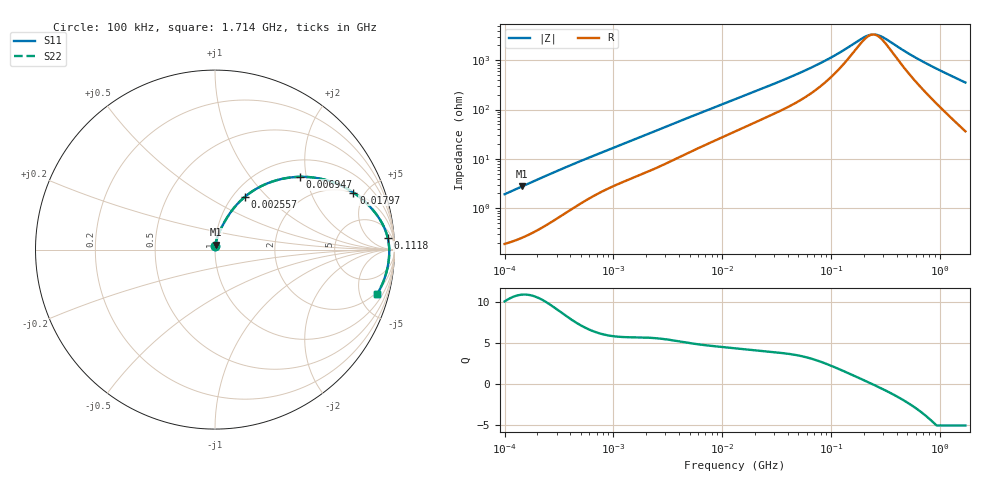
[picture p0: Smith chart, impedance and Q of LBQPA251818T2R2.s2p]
! LBQPA251818T2R2  S-PARAMETER MODEL  ( General Type )
! Model Generated by TAIYO YUDEN Corporation (http://www.ty-top.com)
! Version 1.0
! TAIYO YUDEN Control No. 191025NI43SB-FBB
! Copyright(c) 2019 TAIYO YUDEN CO.,LTD. All Rights Reserved.
! Product Description (link to TY-COMPAS)
! https://ds.yuden.co.jp/TYCOMPAS/or/detail?pn=LBQPA251818T2R2M&u=M
! Products Name : Inductors
! Characteristics :
!  Inductance : 2.2 uH , SRF(min) : 68 MHz , DC Resistance(max) : 0.169 Ohm
!  Rated Current : Saturation :890 mA , Temp Rise : 630 mA (20 degC)
!  Case Size : 2.5 x 1.8 / 0.098 x 0.071 [mm/inch] , Thickness : 1.8 / 0.071 [mm/inch]
!  (Conditions: Temperature = 25 degC , DC Bias Current/Voltage = 0A / 0V)
! External Node Assignments :
!  1  o---GGG---o  2
! GND o---------o GND
! Frequency Range : 0.1MHz  -  1713.942084MHz  [ 402 STEP ]
# MHz S RI R 50
! Freq[MHz].  S11 Real  S11 Imag  S21 Real  S21 Imag  S12 Real  S12 Imag  S22 Real  S22 Imag
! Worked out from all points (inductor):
!   401 points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, 100 kHz to 1.714 GHz, reference 50 ohm
!   read as one part in series: L = 3.04 uH near 105 kHz
!   highest Q = 10.9 at 144.1 kHz (marker M1), where L = 3.04 uH
!   self-resonance near 242.7 MHz
!   S11 on the Smith chart (normalised r, x): 100 kHz: 1.00, +0.04; 2.557 MHz: 1.14, +0.76; 6.947 MHz: 1.38, +1.83; 17.97 MHz: 1.99, +4.15; 111.8 MHz: 13, +23; 1.714 GHz: 1.73, -7.04
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0.1  0.00225 0.0191  0.9977 -0.0191  0.9977 -0.0191  0.00225 0.0191
0.144137  0.00326 0.0274  0.9967 -0.0274  0.9967 -0.0274  0.00326 0.0274
0.511911  0.0208 0.0888  0.9792 -0.0888  0.9792 -0.0888  0.0208 0.0888
1.324369  0.0738 0.1886  0.9262 -0.1886  0.9262 -0.1886  0.0738 0.1886
2.55743  0.1685 0.2957  0.8315 -0.2957  0.8315 -0.2957  0.1685 0.2957
2.620527  0.1736 0.2999  0.8264 -0.2999  0.8264 -0.2999  0.1736 0.2999
4.479799  0.3194 0.3791  0.6806 -0.3791  0.6806 -0.3791  0.3194 0.3791
6.946856  0.4715 0.4055  0.5285 -0.4055  0.5285 -0.4055  0.4715 0.4055
9.536592  0.5842 0.3958  0.4158 -0.3958  0.4158 -0.3958  0.5842 0.3958
13.41476  0.6941 0.3607  0.3059 -0.3607  0.3059 -0.3607  0.6941 0.3607
17.97227  0.7715 0.3176  0.2285 -0.3176  0.2285 -0.3176  0.7715 0.3176
33.05428  0.8815 0.2189  0.1185 -0.2189  0.1185 -0.2189  0.8815 0.2189
67.01815  0.9445 0.1191  0.0555 -0.1191  0.0555 -0.1191  0.9445 0.1191
111.8091  0.9628 0.0638  0.0372 -0.0638  0.0372 -0.0638  0.9628 0.0638
191.138  0.9698 0.0184  0.0302 -0.0184  0.0302 -0.0184  0.9698 0.0184
226.695  0.9707 0.00521  0.0293 -0.00521  0.0293 -0.00521  0.9707 0.00521
268.8666  0.971 -0.00784  0.029 0.00784  0.029 0.00784  0.971 -0.00784
343.0732  0.9706 -0.027  0.0294 0.027  0.0294 0.027  0.9706 -0.027
494.4947  0.9681 -0.0591  0.0319 0.0591  0.0319 0.0591  0.9681 -0.0591
695.5871  0.9623 -0.0956  0.0377 0.0956  0.0377 0.0956  0.9623 -0.0956
1132.534  0.9427 -0.1658  0.0573 0.1658  0.0573 0.1658  0.9427 -0.1658
1713.942  0.9043 -0.2472  0.0957 0.2472  0.0957 0.2472  0.9043 -0.2472
